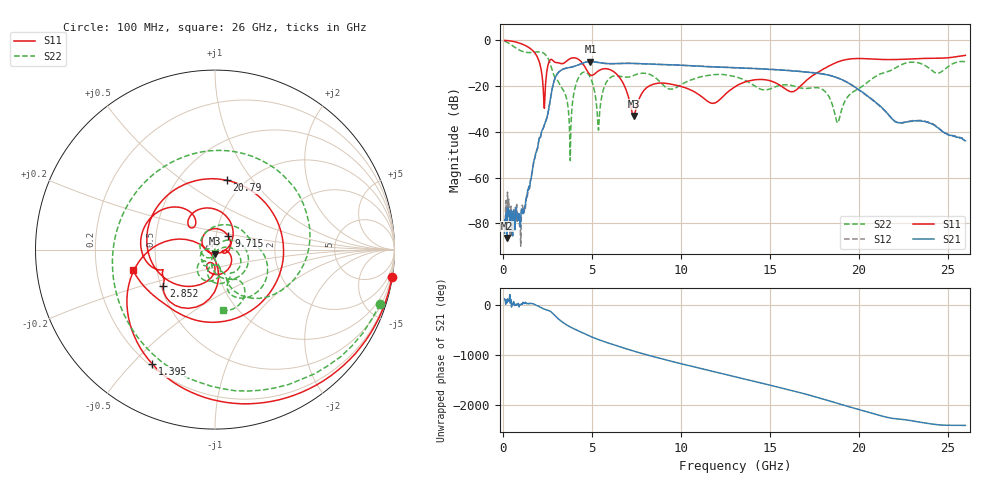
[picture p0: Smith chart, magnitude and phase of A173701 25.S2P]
!  2-Port S-parameters saved by WinCal
! VAR MeasName=S-Parameters (CALIBRATED_DATA) read from VNA (N5245A)
! VAR MeasDate=2017-6-7 10:30:03
! VAR NAME=A173701 25
! VAR FILENAME=A173701 25.S2P
! VAR DATE=2017-6-7 10:30:03
! VAR PHYS_PORTS=1,2
# Hz S DB R 50
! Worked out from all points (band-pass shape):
!   801 points, 100 MHz to 26 GHz, reference 50 ohm
!   highest |S21| = -9.25 dB at 4.924 GHz (marker M1); lowest = -86.5 dB at 229.5 MHz (marker M2)
!   |S21| within 3 dB of the highest: 3.513 GHz to 13.87 GHz (10.35 GHz wide, 119 % of centre)
!   lowest |S11| = -33.1 dB at 7.352 GHz (marker M3), VSWR 1.05, Z = 49.8 - j2.2 ohm
!   |S11| at or under -10 dB: 2.072 GHz to 2.57 GHz (497.9 MHz wide, 21.5 % of centre); 3.21 GHz to 3.418 GHz (208.2 MHz wide, 6.28 % of centre); 4.477 GHz to 18.65 GHz (14.17 GHz wide, 123 % of centre)
!   |S22| runs from -52.6 to -0.3 dB; largest |S21 - S12| = 0.0038
!   S11 on the Smith chart (normalised r, x): 100 MHz: 0, -13; 1.395 GHz: 0.21, -0.57; 2.852 GHz: 0.52, -0.24; 9.715 GHz: 1.15, +0.17; 20.79 GHz: 0.83, +0.75; 26 GHz: 0.36, -0.11
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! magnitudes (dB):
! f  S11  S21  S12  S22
! 100 MHz  0.0  -84.3  -82.3  -0.3
! 229.5 MHz  -0.1  -86.5  -82.6  -0.7
! 941.8 MHz  -1.2  -78.8  -81.1  -4.3
! 1.395 GHz  -2.8  -65.5  -67.3  -5.3
! 1.978 GHz  -7.9  -46.0  -46.2  -5.0
! 2.301 GHz  -26.0  -37.8  -37.8  -5.6
! 2.852 GHz  -9.1  -18.5  -18.5  -14.9
! 3.758 GHz  -8.1  -11.9  -11.8  -41.6
! 4.438 GHz  -9.6  -10.0  -10.1  -14.3
! 4.924 GHz  -15.1  -9.3  -9.3  -16.3
! 5.377 GHz  -13.3  -9.7  -9.7  -39.3
! 5.96 GHz  -12.6  -10.2  -10.2  -16.8
! 7.352 GHz  -33.1  -10.1  -10.1  -15.4
! 8.744 GHz  -18.7  -10.5  -10.5  -17.4
! 9.715 GHz  -19.6  -10.7  -10.8  -20.8
! 11.79 GHz  -27.5  -11.6  -11.5  -15.1
! 13.05 GHz  -20.2  -11.9  -11.9  -15.9
! 17.39 GHz  -15.5  -14.1  -14.0  -20.8
! 18.81 GHz  -9.5  -16.4  -16.4  -36.1
! 20.79 GHz  -8.1  -25.9  -26.2  -16.6
! 21.69 GHz  -8.4  -32.6  -32.7  -13.5
! 26 GHz  -6.5  -43.9  -44.1  -9.3
